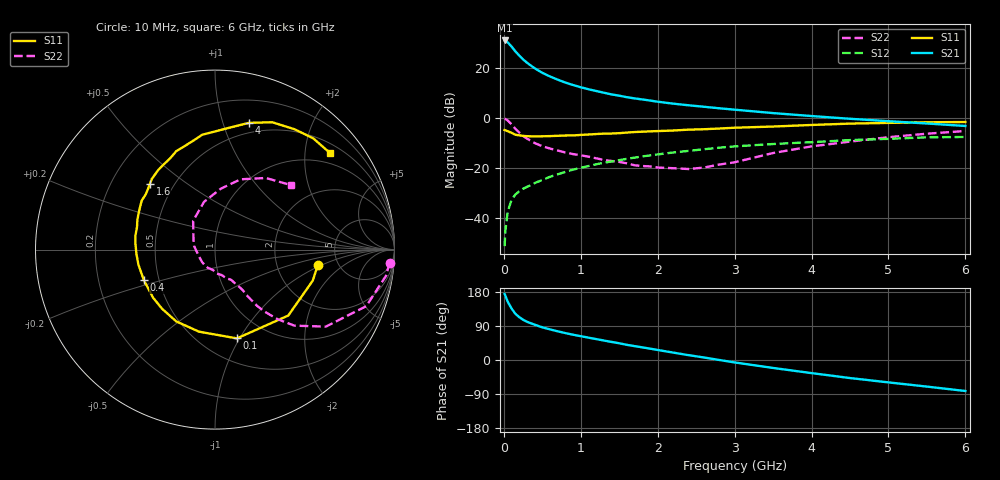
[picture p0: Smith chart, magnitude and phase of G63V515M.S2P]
! SIEMENS Small Signal Semiconductors
! BFG193
! Si NPN RF Bipolar Junction Transistor in SOT223
! VCE = 3.5 V  IC = 15 mA
! Common Emitter S-Parameters:  August  1996
# GHz  S  MA  R  50
!  f  S11  S21  S12  S22
! GHz  MAG  ANG  MAG  ANG  MAG  ANG  MAG  ANG
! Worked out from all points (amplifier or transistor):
!   36 points, 10 MHz to 6 GHz, reference 50 ohm
!   highest |S21| = 31.0 dB at 10 MHz (marker M1)
!   |S21| within 3 dB of that: start of sweep to 115.1 MHz
!   unconditionally stable (mu >= 1): 767.7 MHz to 2.517 GHz
!   at 250 MHz: K = 0.66, MSG = 25.8 dB, |S12| = -28.2 dB
!   at 1.4 GHz: K = 1.06, MAG = 11.9 dB, |S12| = -17.3 dB
!   at 6 GHz: K = 0.88, MSG = 2.2 dB, |S12| = -7.5 dB
!   S11 on the Smith chart (normalised r, x): 10 MHz: 3.49, -0.92; 100 MHz: 0.73, -0.97; 400 MHz: 0.41, -0.17; 1.6 GHz: 0.37, +0.37; 4 GHz: 0.40, +1.22; 6 GHz: 0.71, +2.57
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0.01  0.5789 -8.7  35.39 174.3  0.0028 89.9  0.9754 -4.3
0.02  0.5715 -17.6  35.09 169.6  0.0057 84.1  0.964 -8.7
0.05  0.5492 -42.0  32.5 153.9  0.0136 72.4  0.8998 -20.5
0.1  0.5096 -76.1  26.8 136.0  0.0235 64.2  0.752 -34.8
0.15  0.4659 -101.0  21.43 121.9  0.03 57.6  0.6122 -43.8
0.2  0.4547 -118.3  17.76 113.2  0.0347 56.3  0.5178 -48.2
0.25  0.4422 -131.9  14.87 106.2  0.0391 55.0  0.441 -51.4
0.3  0.4369 -142.2  12.76 100.9  0.0426 55.4  0.3919 -53.2
0.4  0.4313 -156.8  9.882 93.2  0.0506 56.0  0.3191 -55.0
0.5  0.4347 -168.6  8.006 86.2  0.0586 56.4  0.2751 -55.6
0.6  0.4384 -176.7  6.774 80.8  0.0676 56.5  0.2478 -56.9
0.7  0.4442 176.0  5.847 75.7  0.0758 56.9  0.2265 -58.8
0.9  0.452 164.0  4.575 66.7  0.094 55.2  0.1919 -61.7
1.1  0.4715 154.5  3.769 59.0  0.111 53.5  0.1705 -68.7
1.6  0.5158 134.6  2.615 40.0  0.1546 45.4  0.1253 -90.5
2.2  0.566 116.3  1.946 19.6  0.2065 33.7  0.1004 -135.6
2.8  0.6204 100.9  1.573 0.1  0.2575 20.9  0.1187 169.9
3.5  0.68 84.1  1.26 -21.0  0.3049 4.4  0.2016 127.2
4  0.731 75.0  1.102 -34.6  0.3319 -5.2  0.2735 102.8
4.5  0.7779 65.8  0.971 -47.6  0.365 -15.4  0.3403 84.7
5.5  0.827 48.5  0.782 -70.2  0.4144 -39.1  0.4896 54.6
6  0.8366 40.1  0.698 -81.8  0.4211 -52.8  0.5549 40.4
